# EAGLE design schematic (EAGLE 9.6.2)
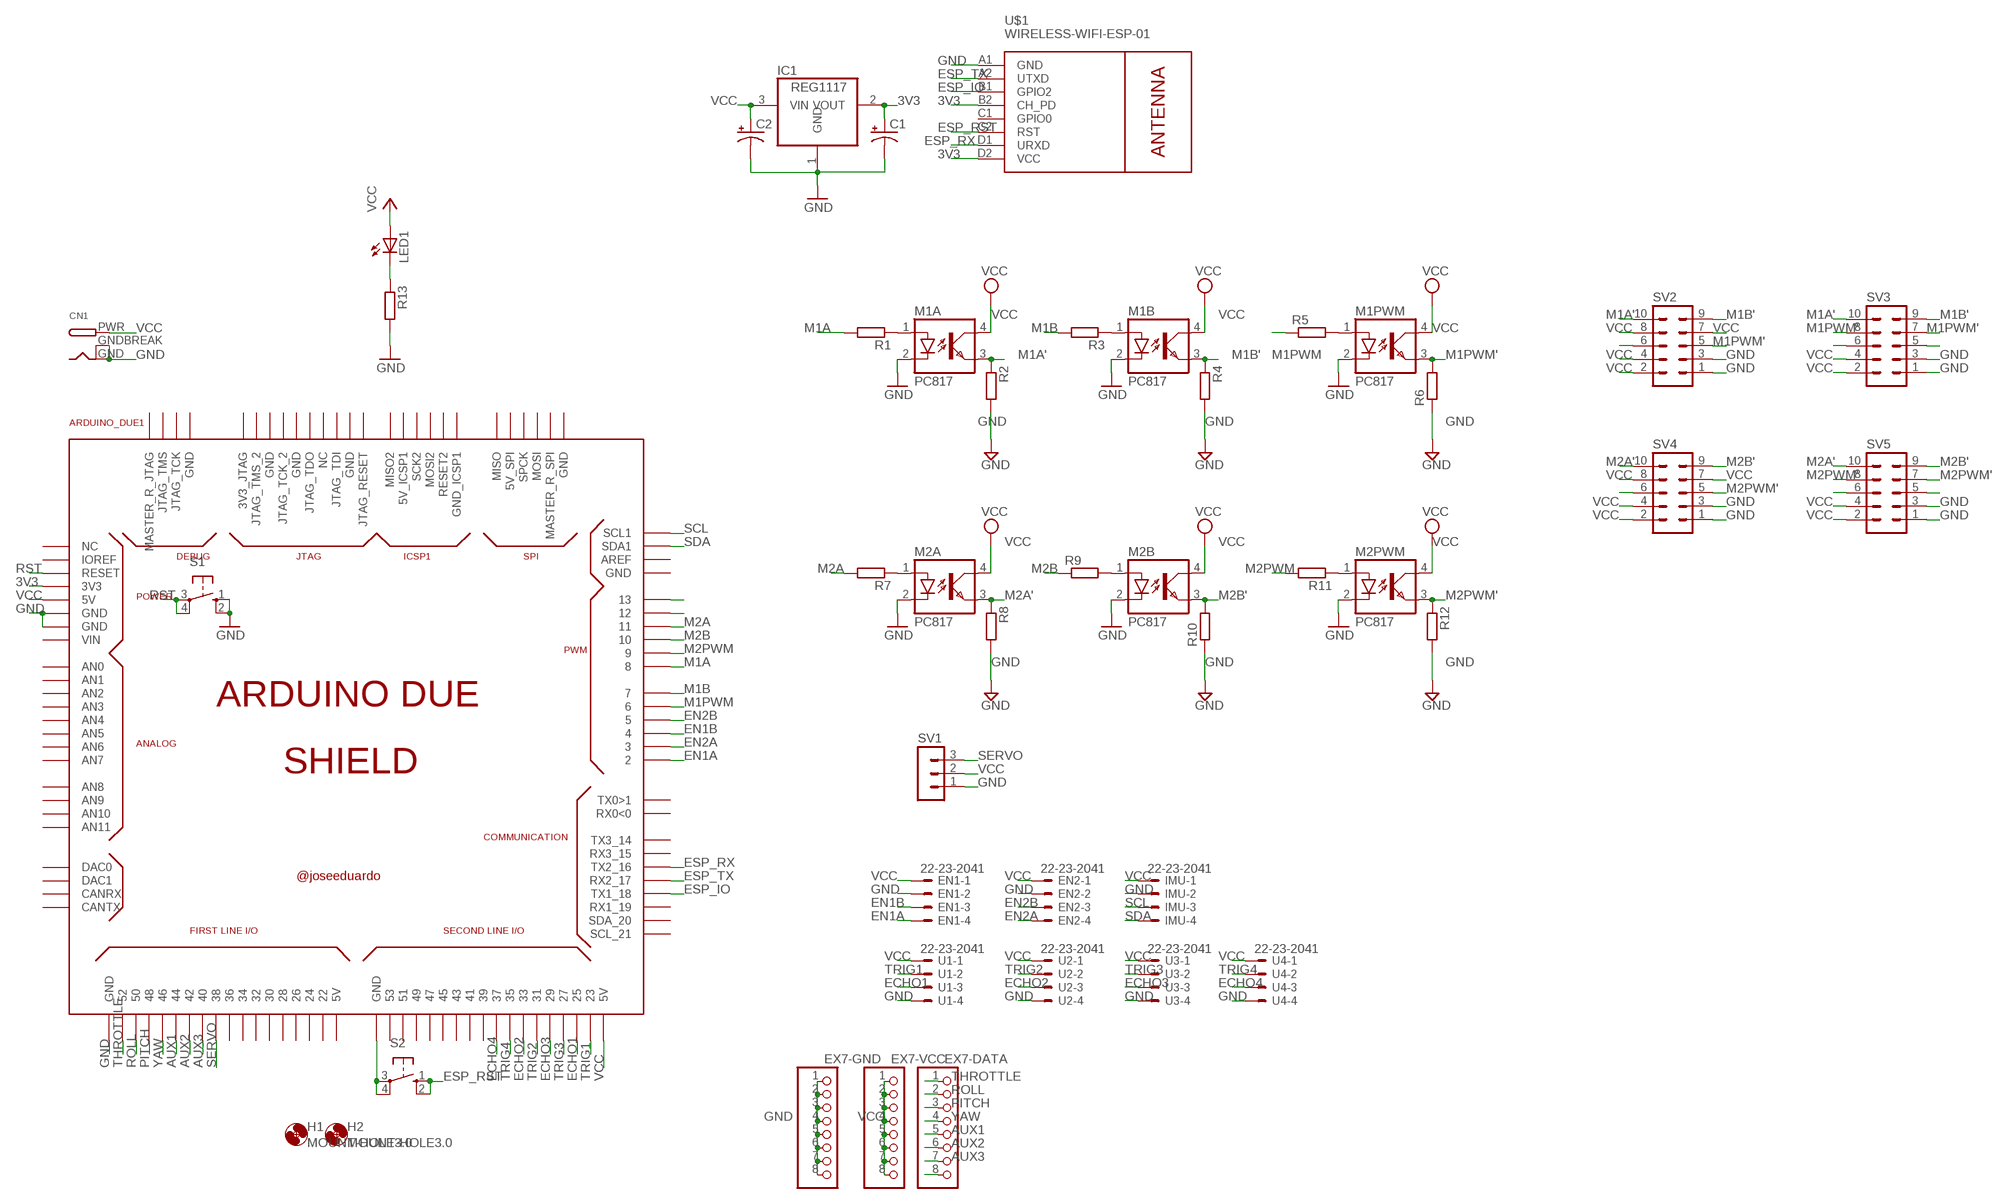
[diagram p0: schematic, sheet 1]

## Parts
ARDUINO_DUE1  ARDUINO_DUE_SHIELD  [ARDUINO_DUE_SHIELD]
C1  CPOL-USTT2D4  [TT2D4]
C2  CPOL-USTT2D4  [TT2D4]
CN1  DCBARRELPTH  [DCJACK_2MM_PTH]
EN1  22-23-2041  [22-23-2041]
EN2  22-23-2041  [22-23-2041]
EX7-DATA  PINHD-1X8BIG  [1X08-BIG]
EX7-GND  PINHD-1X8BIG  [1X08-BIG]
EX7-VCC  PINHD-1X8BIG  [1X08-BIG]
H1  MOUNT-HOLE3.0  [3,0]
H2  MOUNT-HOLE3.0  [3,0]
IC1  REG1117  [SOT223]
IMU  22-23-2041  [22-23-2041]
LED1  LED5MM  [LED5MM]
M1A  PC817  [DIL04]
M1B  PC817  [DIL04]
M1PWM  PC817  [DIL04]
M2A  PC817  [DIL04]
M2B  PC817  [DIL04]
M2PWM  PC817  [DIL04]
R1  R-EU_M0805  [M0805]
R2  R-EU_M0805  [M0805]
R3  R-EU_M0805  [M0805]
R4  R-EU_M0805  [M0805]
R5  R-EU_M0805  [M0805]
R6  R-EU_M0805  [M0805]
R7  R-EU_M0805  [M0805]
R8  R-EU_M0805  [M0805]
R9  R-EU_M0805  [M0805]
R10  R-EU_M0805  [M0805]
R11  R-EU_M0805  [M0805]
R12  R-EU_M0805  [M0805]
R13  R-EU_M0805  [M0805]
S1  40-XX  [B3F-40XX]
S2  40-XX  [B3F-40XX]
SV1  MA03-1  [MA03-1]
SV2  ML10  [ML10]
SV3  ML10  [ML10]
SV4  ML10  [ML10]
SV5  ML10  [ML10]
U1  22-23-2041  [22-23-2041]
U2  22-23-2041  [22-23-2041]
U3  22-23-2041  [22-23-2041]
U4  22-23-2041  [22-23-2041]
U$1  WIRELESS-WIFI-ESP-01  [WIRELESS-WIFI-ESP-01]

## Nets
3V3: ARDUINO_DUE1.3V3 C1.+ IC1.2(VOUT) U$1.B2(CH_PD) U$1.D2(VCC)
AUX1: ARDUINO_DUE1.44 EX7-DATA.5
AUX2: ARDUINO_DUE1.42 EX7-DATA.6
AUX3: ARDUINO_DUE1.40 EX7-DATA.7
ECHO1: ARDUINO_DUE1.25 U1.3
ECHO2: ARDUINO_DUE1.33 U2.3
ECHO3: ARDUINO_DUE1.29 U3.3
ECHO4: ARDUINO_DUE1.37 U4.3
EN1A: ARDUINO_DUE1.2 EN1.4
EN1B: ARDUINO_DUE1.4 EN1.3
EN2A: ARDUINO_DUE1.3 EN2.4
EN2B: ARDUINO_DUE1.5 EN2.3
ESP_IO: ARDUINO_DUE1.18(TX1_18) U$1.B1(GPIO2)
ESP_RST: S2.1(S) S2.2(S1) U$1.C2(RST)
ESP_RX: ARDUINO_DUE1.16(TX2_16) U$1.D1(URXD)
ESP_TX: ARDUINO_DUE1.17(RX2_17) U$1.A2(UTXD)
GND: ARDUINO_DUE1.GND ARDUINO_DUE1.GND_1(GND) ARDUINO_DUE1.GND_2(GND) C1.- C2.- CN1.GND CN1.GNDBREAK EN1.2 EN2.2 EX7-GND.1 EX7-GND.2 EX7-GND.3 EX7-GND.4 EX7-GND.5 EX7-GND.6 EX7-GND.7 EX7-GND.8 IC1.1(GND) IMU.2 M1A.2(C) M1B.2(C) M1PWM.2(C) M2A.2(C) M2B.2(C) M2PWM.2(C) R2.2 R4.2 R6.1 R8.2 R10.1 R12.2 R13.2 S1.1(S) S1.2(S1) SV1.1 SV2.1 SV2.3 SV3.1 SV3.3 SV4.1 SV4.3 SV5.1 SV5.3 U1.4 U2.4 U3.4 U4.4 U$1.A1(GND)
M1A: ARDUINO_DUE1.8 R1.2
M1A': M1A.3(EMIT) R2.1 SV2.10 SV3.10
M1B: ARDUINO_DUE1.7 R3.2
M1B': M1B.3(EMIT) R4.1 SV2.9 SV3.9
M1PWM: ARDUINO_DUE1.6 R5.1
M1PWM': M1PWM.3(EMIT) R6.2 SV2.5 SV3.7 SV3.8
M2A: ARDUINO_DUE1.11 R7.2
M2A': M2A.3(EMIT) R8.1 SV4.10 SV5.10
M2B: ARDUINO_DUE1.10 R9.1
M2B': M2B.3(EMIT) R10.2 SV4.9 SV5.9
M2PWM: ARDUINO_DUE1.9 R11.2
M2PWM': M2PWM.3(EMIT) R12.1 SV4.5 SV5.7 SV5.8
N$1: M1B.1(A) R3.1
N$2: M1A.1(A) R1.1
N$5: M1PWM.1(A) R5.2
N$6: SV2.6
N$7: M2A.1(A) R7.1
N$8: ARDUINO_DUE1.GND_3(GND) S2.3(P) S2.4(P1)
N$9: M2B.1(A) R9.2
N$10: EX7-DATA.8
N$11: M2PWM.1(A) R11.1
N$13: LED1.K(C) R13.1
N$16: ARDUINO_DUE1.12
N$21: ARDUINO_DUE1.13
N$23: SV3.6
N$28: SV3.5
N$33: SV4.6
N$42: SV5.6
N$48: SV5.5
PITCH: ARDUINO_DUE1.48 EX7-DATA.3
ROLL: ARDUINO_DUE1.50 EX7-DATA.2
RST: ARDUINO_DUE1.RESET S1.3(P) S1.4(P1)
SCL: ARDUINO_DUE1.SCL1 IMU.3
SDA: ARDUINO_DUE1.SDA1 IMU.4
SERVO: ARDUINO_DUE1.38 SV1.3
THROTTLE: ARDUINO_DUE1.52 EX7-DATA.1
TRIG1: ARDUINO_DUE1.23 U1.2
TRIG2: ARDUINO_DUE1.31 U2.2
TRIG3: ARDUINO_DUE1.27 U3.2
TRIG4: ARDUINO_DUE1.35 U4.2
VCC: ARDUINO_DUE1.5V0(5V) ARDUINO_DUE1.5V0_2(5V) C2.+ CN1.PWR EN1.1 EN2.1 EX7-VCC.1 EX7-VCC.2 EX7-VCC.3 EX7-VCC.4 EX7-VCC.5 EX7-VCC.6 EX7-VCC.7 EX7-VCC.8 IC1.3(VIN) IMU.1 LED1.A M1A.4(COL) M1B.4(COL) M1PWM.4(COL) M2A.4(COL) M2B.4(COL) M2PWM.4(COL) SV1.2 SV2.2 SV2.4 SV2.7 SV2.8 SV3.2 SV3.4 SV4.2 SV4.4 SV4.7 SV4.8 SV5.2 SV5.4 U1.1 U2.1 U3.1 U4.1
YAW: ARDUINO_DUE1.46 EX7-DATA.4
Unconnected: ARDUINO_DUE1.0(RX0<0) ARDUINO_DUE1.1(TX0>1) ARDUINO_DUE1.3V3_JTAG ARDUINO_DUE1.5V0_1(5V) ARDUINO_DUE1.5V_2(5V_SPI) ARDUINO_DUE1.5V_ICSP1 ARDUINO_DUE1.14(TX3_14) ARDUINO_DUE1.15(RX3_15) ARDUINO_DUE1.19(RX1_19) ARDUINO_DUE1.20(SDA_20) ARDUINO_DUE1.21(SCL_21) ARDUINO_DUE1.22 ARDUINO_DUE1.24 ARDUINO_DUE1.26 ARDUINO_DUE1.28 ARDUINO_DUE1.30 ARDUINO_DUE1.32 ARDUINO_DUE1.34 ARDUINO_DUE1.36 ARDUINO_DUE1.39 ARDUINO_DUE1.41 ARDUINO_DUE1.43 ARDUINO_DUE1.45 ARDUINO_DUE1.47 ARDUINO_DUE1.49 ARDUINO_DUE1.51 ARDUINO_DUE1.53 ARDUINO_DUE1.A0(AN0) ARDUINO_DUE1.A1(AN1) ARDUINO_DUE1.A2(AN2) ARDUINO_DUE1.A3(AN3) ARDUINO_DUE1.A4(AN4) ARDUINO_DUE1.A5(AN5) ARDUINO_DUE1.A6(AN6) ARDUINO_DUE1.A7(AN7) ARDUINO_DUE1.A8(AN8) ARDUINO_DUE1.A9(AN9) ARDUINO_DUE1.A10(AN10) ARDUINO_DUE1.A11(AN11) ARDUINO_DUE1.AREF ARDUINO_DUE1.CANRX ARDUINO_DUE1.CANTX ARDUINO_DUE1.DAC0 ARDUINO_DUE1.DAC1 ARDUINO_DUE1.GND_4(GND) ARDUINO_DUE1.GND_5(GND) ARDUINO_DUE1.GND_7(GND) ARDUINO_DUE1.GND_8(GND) ARDUINO_DUE1.GND_9(GND) ARDUINO_DUE1.GND_10(GND) ARDUINO_DUE1.GND_ICSP1 ARDUINO_DUE1.IOREF ARDUINO_DUE1.JTAG_RESET ARDUINO_DUE1.JTAG_TCK ARDUINO_DUE1.JTAG_TCK_2 ARDUINO_DUE1.JTAG_TDI ARDUINO_DUE1.JTAG_TDO ARDUINO_DUE1.JTAG_TMS ARDUINO_DUE1.JTAG_TMS_2 ARDUINO_DUE1.MASTER_RESET_JTAG(MASTER_R_JTAG) ARDUINO_DUE1.MASTER_RESET_SPI(MASTER_R_SPI) ARDUINO_DUE1.MISO ARDUINO_DUE1.MISO2 ARDUINO_DUE1.MOSI ARDUINO_DUE1.MOSI2 ARDUINO_DUE1.NC_2(NC) ARDUINO_DUE1.NC_5(NC) ARDUINO_DUE1.RESET2 ARDUINO_DUE1.SCK2 ARDUINO_DUE1.SPCK ARDUINO_DUE1.VIN U$1.C1(GPIO0)

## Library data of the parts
ARDUINO_DUE1 = arduino_due_shield:ARDUINO_DUE_SHIELD
C1 C2 = adafruit:CPOL-US: POLARIZED CAPACITOR, American symbol
CN1 = adafruit:DCBARREL: 2.0mm DC Barrel Jack DCJACK_2MM_PTH - Through Hole Jack (4UConnector: 05537)
EN1 EN2 IMU U1-U4 = con-molex:22-23-2041: .100" (2.54mm) Center Header - 4 Pin; MF: MOLEX; MPN: 22-23-2041; OC_FARNELL: 1462920; OC_NEWARK: 38C0355
EX7-DATA EX7-GND EX7-VCC = adafruit:PINHD-1X8: PIN HEADER
H1 H2 = holes:MOUNT-HOLE: MOUNTING HOLE with drill center marker
IC1 = burr-brown:REG1117: 800mA and 1A Low Dropout (LDO) Positive Regulator 1.8V, 2.5V, 2.85V, 3.3V, 5V, and Adj; MPN: REG1117; OC_FARNELL: 1097566; OC_NEWARK: 14P6981
LED1 = adafruit:LED: LED
M1A M1B M1PWM M2A M2B M2PWM = optocoupler:PC817: SHARP OPTO COUPLER; MPN: PC817X4J000F; OC_FARNELL: 9707727; OC_NEWARK: 97K7059
R1-R13 = rcl:R-EU_: RESISTOR, European symbol; SPICEPREFIX: R
S1 S2 = adafruit:40-XX: OMRON SWITCH; MF: OMRON COMPONENTS USA; MPN: B3F-4000; OC_FARNELL: 176434; OC_NEWARK: 36K3105
SV1 = con-lstb:MA03-1: PIN HEADER; OC_FARNELL: unknown; OC_NEWARK: unknown
SV2-SV5 = con-ml:ML10: HARTING; OC_FARNELL: unknown; OC_NEWARK: unknown
U$1 = ESP-01:WIRELESS-WIFI-ESP-01: Wireless Wi-Fi ESP-01 Module based on ESP8266 chip Click here to find device on ebay.com

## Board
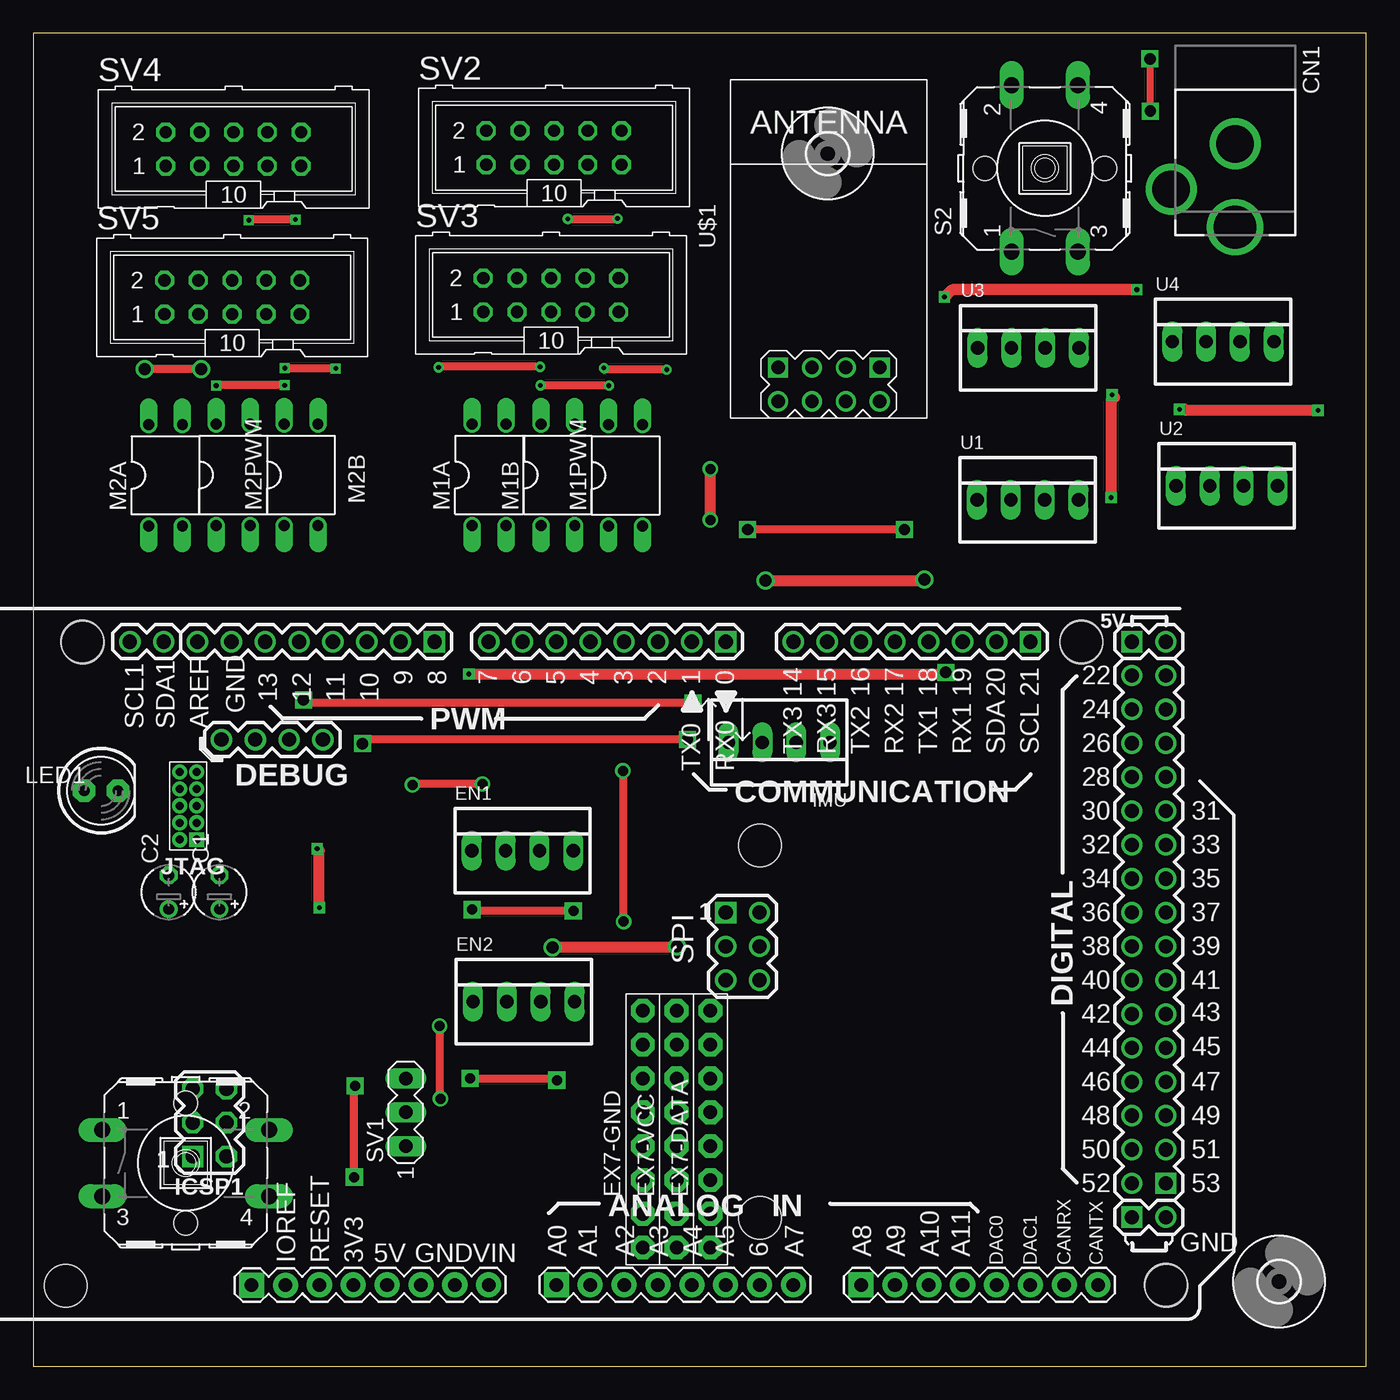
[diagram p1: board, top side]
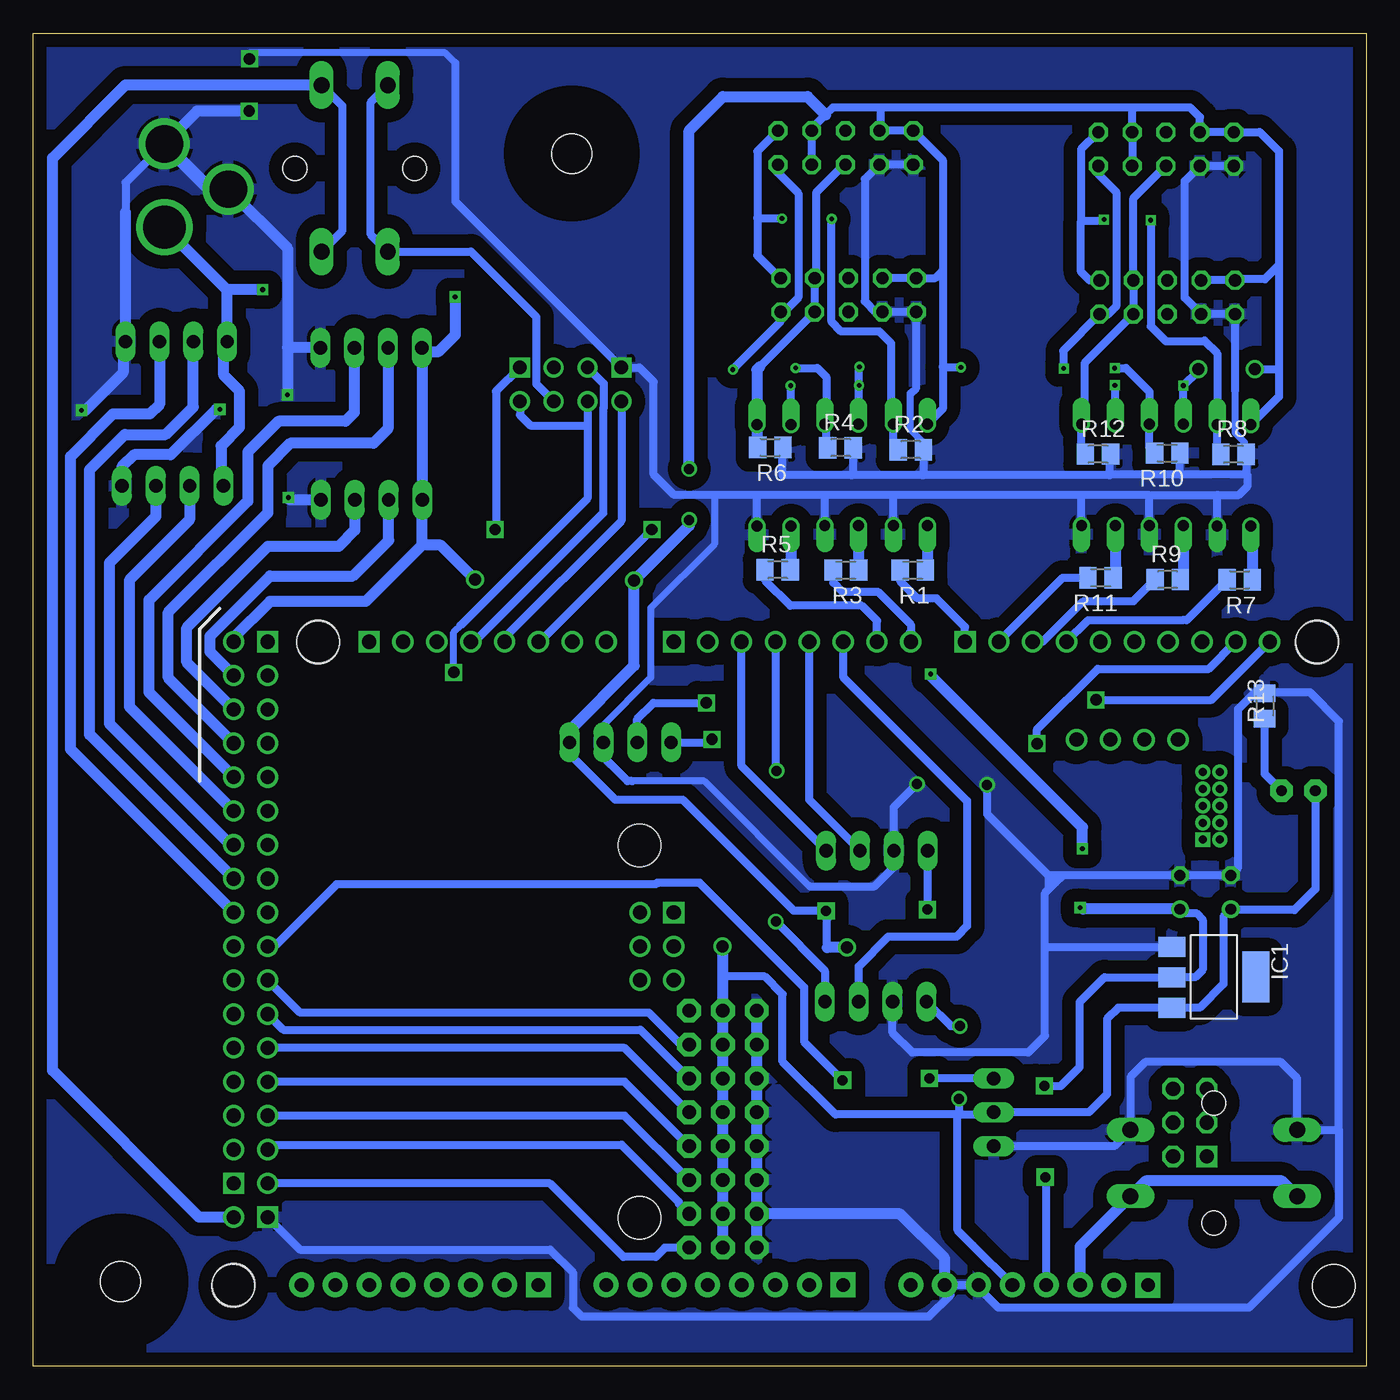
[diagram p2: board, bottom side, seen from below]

Size 100 x 100 mm. Coordinates in mm from the lower left corner, seen from the top.
Outline: 0,0 100,0 100,100 0,100 0,0
Copper layers (1*16): Top 0.035mm / dielectric 1.5mm / Bottom 0.035mm
Design rules "default": minimum track width 6mil, minimum drill 0.35mm, track to track 6mil, track to pad 6mil, pad to pad 6mil, via to via 6mil, smd to smd 6mil, copper to edge 40mil, drill to drill 6mil, minimum pad ring 10mil, minimum via ring 8mil, stop-mask expansion 4mil, vias tented up to drill 0mil, thermal gap 10mil

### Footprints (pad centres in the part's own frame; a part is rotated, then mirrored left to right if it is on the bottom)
ARDUINO_DUE_SHIELD = drill 1.067 square: 0 63.373,51.816; 5V0_1 93.853,51.816; 8 41.529,51.816; 21 86.233,51.816; 53 96.393,11.176; GND_2 93.853,8.636; MISO 63.373,31.496; MISO2 23.384,13.196 | drill 1.067: 1 60.833,51.816; 2 58.293,51.816; 3 55.753,51.816; 4 53.213,51.816; 5 50.673,51.816; 5V0_2 96.393,51.816; 5V_2 65.913,31.496; 6 48.133,51.816; 7 45.593,51.816; 9 38.989,51.816; 10 36.449,51.816; 11 33.909,51.816; 12 31.369,51.816; 13 28.829,51.816; 14 68.453,51.816; 15 70.993,51.816; 16 73.533,51.816; 17 76.073,51.816; 18 78.613,51.816; 19 81.153,51.816; 20 83.693,51.816; 22 93.853,49.276; 23 96.393,49.276; 24 93.853,46.736; 25 96.393,46.736; 26 93.853,44.196; 27 96.393,44.196; 28 93.853,41.656; 29 96.393,41.656; 30 93.853,39.116; 31 96.393,39.116; 32 93.853,36.576; 33 96.393,36.576; 34 93.853,34.036; 35 96.393,34.036; 36 93.853,31.496; 37 96.393,31.496; 38 93.853,28.956; 39 96.393,28.956; 40 93.853,26.416; 41 96.393,26.416; 42 93.853,23.876; 43 96.393,23.876; 44 93.853,21.336; 45 96.393,21.336; 46 93.853,18.796; 47 96.393,18.796; 48 93.853,16.256; 49 96.393,16.256; 50 93.853,13.716; 51 96.393,13.716; 52 93.853,11.176; AREF 23.749,51.816; GND_3 96.393,8.636; GND_4 26.289,51.816; GND_5 65.913,26.416; GND_7 33.161,44.473; JTAG_TCK 30.621,44.473; JTAG_TMS 28.081,44.473; MASTER_RESET_JTAG 25.541,44.473; MASTER_RESET_SPI 63.373,26.416; MOSI 65.913,28.956; SCL1 18.669,51.816; SDA1 21.209,51.816; SPCK 63.373,28.956 | drill 1.016 pad 1.88: 3V3 35.433,3.556; 5V0 37.973,3.556; A1 53.213,3.556; A2 55.753,3.556; A3 58.293,3.556; A4 60.833,3.556; A5 63.373,3.556; A6 65.913,3.556; A7 68.453,3.556; A9 76.073,3.556; A10 78.613,3.556; A11 81.153,3.556; CANRX 88.773,3.556; CANTX 91.313,3.556; DAC0 83.693,3.556; DAC1 86.233,3.556; GND 40.513,3.556; GND_1 43.053,3.556; IOREF 30.346,3.543; RESET 32.893,3.555; VIN 45.593,3.556 | drill 0.6 pad 1.016 square: 3V3_JTAG 23.689,36.964 | drill 1.067 octagon: 5V_ICSP1 25.924,13.196; GND_ICSP1 25.924,18.276; MOSI2 25.924,15.736; RESET2 23.384,18.276; SCK2 23.384,15.736 | drill 1.016 pad 1.88 square: A0 50.673,3.556; A8 73.533,3.556; NC_2 27.806,3.543 | drill 0.6 pad 1.143: GND_8 23.689,38.234; GND_9 23.689,40.774; GND_10 23.689,42.044; JTAG_RESET 22.419,42.044; JTAG_TCK_2 22.419,38.234; JTAG_TDI 22.419,40.774; JTAG_TDO 22.419,39.504; JTAG_TMS_2 22.419,36.964; NC_5 23.689,39.504 | hole 3.2: 15.113,51.816; 90.043,51.816; 96.393,3.556; 96.418,3.505; 15.138,51.765; 90.068,51.765; 13.868,3.505; 65.938,36.525; 65.938,8.585
TT2D4 = drill 0.813: + -1.27,0 | drill 0.813 octagon: - 1.27,0
DCJACK_2MM_PTH = drill 2.8: GND 0,7.35; GNDBREAK 4.8,10.75 | drill 3.2: PWR 0,13.6
22-23-2041 = drill 1 long: 1 -3.81,0; 2 -1.27,0; 3 1.27,0; 4 3.81,0
1X08-BIG = drill 1.016 pad 1.778 octagon: 1 -8.89,0; 2 -6.35,0; 3 -3.81,0; 4 -1.27,0; 5 1.27,0; 6 3.81,0; 7 6.35,0; 8 8.89,0
3,0 = hole 3: 0,0
SOT223 = smd 1.499 x 2.007: 1 -2.261,-3.15; 2 0.025,-3.15; 3 2.311,-3.15 | smd 3.81 x 2.007: 4 0,3.15
LED5MM = drill 0.813 pad 1.676 octagon: A -1.27,0; K 1.27,0
DIL04 = drill 0.813 offset: 1 -1.27,-3.81; 2 1.27,-3.81; 3 1.27,3.81; 4 -1.27,3.81
M0805 = smd 1.3 x 1.6: 1 -0.95,0; 2 0.95,0
B3F-40XX = drill 1.194 long: 1 -6.248,2.489; 2 6.248,2.489; 3 -6.248,-2.489; 4 6.248,-2.489 | hole 1.803: 0,-4.496; 0,4.496
MA03-1 = drill 1.016 long: 1 -2.54,0; 2 0,0; 3 2.54,0
ML10 = drill 0.914 octagon: 1 -5.08,-1.27; 2 -5.08,1.27; 3 -2.54,-1.27; 4 -2.54,1.27; 5 0,-1.27; 6 0,1.27; 7 2.54,-1.27; 8 2.54,1.27; 9 5.08,-1.27; 10 5.08,1.27
WIRELESS-WIFI-ESP-01 = drill 1 square: A1 -8.89,3.81; D1 -8.89,-3.81 | drill 1: A2 -11.43,3.81; B1 -8.89,1.27; B2 -11.43,1.27; C1 -8.89,-1.27; C2 -11.43,-1.27; D2 -11.43,-3.81

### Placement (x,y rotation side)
ARDUINO_DUE1  -11.43,2.54 0 top
C1  13.97,35.56 90 top
C2  10.16,35.56 90 top
CN1  90.17,99.06 180 top
EN1  36.71,38.68 0 top
EN2  36.8,27.35 0 top
EX7-DATA  50.8,17.78 90 top
EX7-GND  45.72,17.78 90 top
EX7-VCC  48.26,17.78 90 top
H1  93.46,6.35 0 top
H2  59.61,90.97 0 top
IC1  11.43,29.21 270 bottom
IMU  55.96,46.8 180 top
LED1  5.08,43.18 0 top
M1A  34.19,66.87 0 top
M1B  39.35,66.87 0 top
M1PWM  44.44,66.83 0 top
M2A  9.92,66.84 0 top
M2B  14.99,66.87 0 top
M2PWM  20.08,66.87 0 top
R1  34.02,59.73 180 bottom
R2  34.17,68.76 0 bottom
R3  39.04,59.73 180 bottom
R4  39.44,68.91 0 bottom
R5  44.15,59.75 0 bottom
R6  44.7,68.93 180 bottom
R7  9.5,58.99 180 bottom
R8  9.95,68.41 0 bottom
R9  14.9,59.02 0 bottom
R10  14.94,68.51 180 bottom
R11  19.93,59.16 180 bottom
R12  20.12,68.43 0 bottom
R13  7.62,49.53 90 bottom
S1  11.43,15.24 0 top
S2  75.89,89.87 90 top
SV1  27.94,19.05 90 top
SV2  39.06,91.42 0 top
SV3  38.84,80.37 0 top
SV4  15.02,91.32 0 top
SV5  14.92,80.19 0 top
U1  74.61,64.99 0 top
U2  89.54,66.04 0 top
U3  74.65,76.41 0 top
U4  89.27,76.87 0 top
U$1  59.69,83.82 90 top

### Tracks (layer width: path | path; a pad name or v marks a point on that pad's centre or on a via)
3V3  (via drill 0.35 pad 0.85, 0.75 pad 1.3, 0.85 pad 0.85)
  Top 0.61: v24.08,14.18 24.08,20.72 23.96,20.84 v24.14,21.02
  Top 0.813: v21.45,34.39 21.45,38.66 v21.29,38.82 | v21.29,38.82 | v32.68,51.93 68.56,51.93 68.57,51.95 v68.45,52.06
  Bottom 0.508: v68.45,52.06 68.45,55.08 67.96,55.57
  Bottom 0.61: C1.+ 13.67,33.99 12.76,33.99 12.26,33.49 12.26,29.75 12.82,29.18 IC1.2 19.63,29.18 21.5,27.32 21.5,22.44 22.91,21.02 v24.14,21.02 | U$1.D2 63.5,71.36 62.71,70.57 58.57,70.57 58.42,70.72 | ARDUINO_DUE1.3V3 24,14.1 v24.08,14.18 | 58.42,70.72 58.42,65.11 67.96,55.57 | U$1.B2 58.42,70.72
  Bottom 0.813: C1.+ 21.24,34.29 21.4,34.44 v21.45,34.39 | v21.29,38.82 21.29,40.44 32.68,51.83 v32.68,51.93
AUX1
  Bottom 0.61: EX7-DATA.5 55.63,23.88 ARDUINO_DUE1.44
AUX2
  Bottom 0.61: EX7-DATA.6 54.45,25.24 81.25,25.24 ARDUINO_DUE1.42
AUX3
  Bottom 0.61: EX7-DATA.7 51.44,24.13 53.82,26.51 79.98,26.51 ARDUINO_DUE1.40
ECHO1
  Bottom 0.813: ARDUINO_DUE1.25 88.49,52.81 88.49,55.42 82.4,61.51 77.09,61.51 75.88,62.72 U1.3
ECHO2
  Bottom 0.813: U2.3 90.81,63.76 94.3,60.27 94.3,48.22 85.2,39.12 ARDUINO_DUE1.33
ECHO3
  Bottom 0.813: ARDUINO_DUE1.29 91.31,50.54 91.31,57.49 83.92,64.89 83.92,68.58 81.61,70.89 76.58,70.89 75.92,71.55 U3.3
ECHO4
  Bottom 0.813: ARDUINO_DUE1.37 97.2,46.28 97.2,68.26 94.03,71.43 91.25,71.43 90.54,72.15 U4.3
EN1A
  Bottom 0.61: EN1.4 46.86,45.03 ARDUINO_DUE1.2
EN1B
  Bottom 0.61: EN1.3 41.78,42.49 ARDUINO_DUE1.4
EN2A  (via drill 0.75)
  Top 0.61: v44.23,44.66 44.23,33.42 v44.29,33.36
  Bottom 0.61: ARDUINO_DUE1.3 44.32,44.75 v44.23,44.66 | v44.29,33.36 40.61,29.67 EN2.4
EN2B
  Bottom 0.61: ARDUINO_DUE1.5 39.24,51.72 29.94,42.42 29.94,33.01 30.72,32.23 35.85,32.23 38.07,30.01 EN2.3
ESP_IO
  Bottom 0.61: U$1.B1 57.21,73.72 57.21,71.89 57.24,71.86 57.24,64 66.89,54.36 ARDUINO_DUE1.18
ESP_RST
  Bottom 0.61: U$1.C2 62.27,73.7 62.27,78.74 67.16,83.62 S2.1 74.69,84.91 74.69,94.83 S2.2
ESP_RX  (via drill 0.85 pad 0.85)
  Top 0.61: v65.35,62.77 54.02,62.77 53.96,62.83 53.65,62.83 v53.59,62.77
  Bottom 0.61: U$1.D1 65.29,73.14 65.29,62.83 v65.35,62.77 | v53.59,62.77 62,54.36 ARDUINO_DUE1.16
ESP_TX
  Bottom 0.61: U$1.A2 55.88,63.42 64.64,54.65 ARDUINO_DUE1.17
GND  (via drill 0.35 pad 0.85, 0.75, 0.85 pad 0.85)
  Top 0.508: v83.78,98.08 83.78,94.33 83.87,94.24 v83.81,94.17
  Top 0.61: v33.7,43.68 28.52,43.68 v28.45,43.61
  Top 0.813: v96.4,71.71 86.48,71.71 86.42,71.77 86.01,71.77 v85.99,71.78 | v80.88,65.17 80.88,72.45 81.12,72.69 | 81.12,72.69 | 81.12,72.69 v80.94,72.88
  Bottom 0.152: 36.39,79.1 SV3.3
  Bottom 0.508: 48.91,65.36 48.91,61.65 53.67,56.88 53.67,51.66 57.23,48.1 IMU.2 | 41.75,36.01 49.65,43.9 55.07,43.9 | 68.34,97.79 69.09,98.53 83.78,98.53 v83.78,98.08 | R2.2 33.22,69.3 34.2,70.27 34.2,72.96 34.18,72.98 | 9.84,73.2 9.84,70.03 9.13,69.32 9.13,68.54 R8.2
  Bottom 0.61: 7.99,50.48 8.44,50.48 9.6,49.32 9.6,37.39 C2.- C1.- 22.77,36.83 | 7.99,50.48 R13.2 | SV1.1 18.9,16.51 S1.2 17.68,21.7 16.57,22.81 6.41,22.81 5.18,21.59 S1.1 2.04,17.73 | ARDUINO_DUE1.GND_1 31.19,6.1 | 31.19,6.1 ARDUINO_DUE1.GND 29.08,5.89 27.61,4.42 8.78,4.42 2.03,11.16 2.03,17.72 2.04,17.73 | 2.04,17.73 2.04,48.39 4.2,50.55 7.92,50.55 7.99,50.48 | IC1.1 24.06,31.47 24.1,31.51 | ARDUINO_DUE1.GND_2 80,8.75 61.21,8.75 59.51,7.04 59.51,4.38 58.87,3.73 32.79,3.73 31.19,5.33 31.19,6.1 | 24.1,31.51 24.1,24.8 25.36,23.54 34.06,23.54 35.53,25.01 EN2.2 | 24.1,31.51 24.1,35.5 23.85,35.75 | 23.85,35.75 23.31,36.29 | 23.31,36.29 22.77,36.83 | M2A.2 11.19,65.34 11.16,65.36 | 16.36,65.36 11.16,65.36 | 16.36,65.36 21.42,65.36 | 21.42,65.36 35.33,65.36 | 35.33,65.36 40.65,65.36 | 40.65,65.36 45.71,65.36 | M1PWM.2 45.71,65.36 | M2B.2 16.26,65.26 16.36,65.36 | M2PWM.2 21.35,65.3 21.42,65.36 | M1A.2 35.46,65.23 35.33,65.36 | M1B.2 40.62,65.34 40.65,65.36 | 45.71,65.36 48.91,65.36 51.93,65.36 53.47,66.9 53.47,73.87 54.53,74.93 U$1.A1 68.34,87.39 68.34,97.79 | CN1.GND 90.41,91.47 93.08,88.8 93.08,86.55 | 55.07,43.9 55.43,43.9 57.23,45.71 IMU.2 | R8.2 9,66.96 | 9,66.96 9.09,66.88 13.87,66.88 | R10.1 13.99,67 13.87,66.88 | 13.87,66.88 19.18,66.88 19.24,66.82 19.24,66.85 | 19.24,66.85 19.24,68.35 R12.2 | 19.24,66.85 33.27,66.85 | 33.27,66.85 33.25,66.82 33.22,66.85 R2.2 | 33.27,66.85 38.61,66.85 | 38.61,66.85 43.73,66.85 43.78,66.8 43.78,68.9 R6.1 | R4.2 38.49,66.96 38.61,66.85 | SV3.3 SV3.1 33.76,73.4 34.18,72.98 | SV2.1 SV2.3 37.61,89.07 37.61,79.9 36.8,79.1 36.39,79.1 | SV4.1 SV4.3 13.61,88.91 13.61,80.16 SV5.3 SV5.1 9.84,73.2
  Bottom 0.61: 11.16,65.36 9.57,65.36 8.89,66.04 8.89,66.85 9,66.96 | 41.75,36.01 36.88,36.01 35.44,37.44 EN1.2 35.44,41.95 v33.7,43.68 | v28.45,43.61 28.45,41.43 23.85,36.83 | 23.85,36.83 23.31,36.29 | 22.77,36.83 23.85,36.83 | 23.85,36.83 23.85,35.75
  Bottom 0.813: U2.4 93.35,67.48 92.45,68.39 89.7,68.39 86.3,71.78 v85.99,71.78 | v96.4,71.71 96.09,71.71 93.26,74.53 93.26,76.69 U4.4 93.08,86.55 | U1.4 80.76,64.99 80.88,65.11 v80.88,65.17 | CN1.GNDBREAK 80.94,83.88 80.94,76.46 | 80.94,76.46 v80.94,72.88 | U3.4 80.89,76.41 80.94,76.46 | v83.81,94.17 87.71,94.17 90.41,91.47 | EX7-GND.1 EX7-GND.2 | EX7-GND.2 EX7-GND.3 EX7-GND.4 EX7-GND.5 EX7-GND.6 EX7-GND.7 EX7-GND.8 | ARDUINO_DUE1.GND_1 31.62,8.09 34.97,11.43 EX7-GND.2
  Bottom 1.016: CN1.GND 86.77,88.31 CN1.GNDBREAK
  pour Bottom (isolate 1.016): 0,99.06 0,0 100.33,0 100.33,100.33 0,100.33
M1A
  Bottom 0.61: R1.2 34.97,58.92 33.65,57.6 32.23,57.6 30.1,55.47 ARDUINO_DUE1.8
M1A'  (via drill 0.35)
  Top 0.61: v40.1,86.07 43.78,86.07 43.81,86.1 v43.84,86.1
  Bottom 0.152: SV2.10 44.33,92.5
  Bottom 0.61: 45.68,86.16 45.68,91.16 44.33,92.5 | 45.68,86.16 45.68,83.33 43.99,81.64 SV3.10 | v43.84,86.1 45.62,86.1 45.68,86.16 | v40.1,86.07 40.12,86.06 40.12,78.36 39.39,77.63 36.52,77.63 35.63,76.73 35.63,70.85 M1A.3 35.46,69.09 R2.1
M1B
  Bottom 0.61: R3.2 39.99,58.78 39.32,58.11 36.64,58.11 34.16,55.63 34.16,54.94
  Bottom 0.813: 34.16,54.94 ARDUINO_DUE1.7
M1B'  (via drill 0.35)
  Top 0.61: v47.52,74.77 42.85,74.77 42.77,74.85 v42.81,74.89
  Bottom 0.152: 43.53,79.24 43.67,79.1 SV3.9
  Bottom 0.61: 43.53,79.24 42.6,80.17 42.6,87.99 44.14,89.54 SV2.9 | SV3.9 43.92,78.42 47.52,74.82 v47.52,74.77 | v42.81,74.89 41.19,74.89 40.5,74.21 40.5,70.8 | 40.5,70.8 M1B.3 | R4.1 40.5,69.02 40.5,70.8
M1PWM
  Bottom 0.61: R5.1 45.1,58.96 43.21,57.06 37.84,57.06 36.7,55.93 ARDUINO_DUE1.6
M1PWM'
  Bottom 0.152: 41.41,81.66 SV3.8 41.38,81.94
  Bottom 0.61: SV3.8 SV3.7 45.48,74.99 | SV2.5 39.16,90.16 41.28,88.04 41.28,82.05 41.38,81.94
  Bottom 0.813: 45.48,74.99 45.71,74.77 45.71,71.14 | 45.71,71.14 M1PWM.3 | R6.2 45.65,71.08 45.71,71.14
M2A
  Bottom 0.61: ARDUINO_DUE1.11 20.86,55.98 13.78,55.98 13.46,55.98 R7.2
M2A'  (via drill 0.35)
  Top 0.61: v19.68,86.03 16.17,86.03 v16.17,85.99
  Bottom 0.152: 20.04,81.47 SV5.10
  Bottom 0.61: SV4.10 21.4,91.29 21.4,85.9 | 21.4,85.9 21.4,82.11 20.76,81.47 20.04,81.47 | 21.4,85.9 21.36,85.94 19.74,85.94 19.68,86.01 v19.68,86.03 | v16.17,85.99 16.17,78.03 15.03,76.89 12.2,76.89 12.13,76.95 11.19,76 M2A.3 11.19,68.69 R8.1
M2B
  Bottom 0.61: R9.1 17.46,57.4 21.21,57.4 24.26,54.36 ARDUINO_DUE1.10
M2B'  (via drill 0.35)
  Top 0.61: v22.69,74.85 18.9,74.85 v18.86,74.89
  Bottom 0.152: 18.94,79.33 18.88,79.39
  Bottom 0.61: 18.88,79.39 18.75,79.53 18.75,88.08 20.1,89.44 SV4.9 | 18.94,79.33 19.35,78.92 SV5.9 22.74,76.19 22.74,74.82 22.69,74.82 v22.69,74.85 | v18.86,74.89 18.03,74.89 16.26,73.11 M2B.3 16.26,68.88 R10.2
M2PWM
  Bottom 0.61: ARDUINO_DUE1.9 22.76,59.16 R11.2
M2PWM'
  Bottom 0.61: SV4.5 15.06,90.05 17.46,87.64 SV5.8 SV5.7 21.13,75.26 21.13,70.9 M2PWM.3 21.35,68.7 R12.1
N$1
  Bottom 0.813: M1B.1 38.08,60.03 38.09,60.02 R3.1
N$2
  Bottom 0.813: M1A.1 32.92,59.9 33.07,59.75 R1.1
N$5
  Bottom 0.813: M1PWM.1 43.17,60.49 R5.2
N$7
  Bottom 0.813: M2A.1 8.56,62.95 8.56,59 R7.1
N$8
  Bottom 0.61: S2.4 76.8,94.53 76.8,85.2 S2.3
  Bottom 0.813: 78.32,96.06 S2.4 93.09,96.12 98.56,90.65 98.56,22.18 87.56,11.18 ARDUINO_DUE1.GND_3
N$9
  Bottom 0.813: M2B.1 13.72,59.24 R9.2
N$11
  Bottom 0.813: M2PWM.1 18.81,59.32 R11.1
N$13
  Bottom 0.61: LED1.K 7.62,44.45 R13.1
PITCH
  Bottom 0.61: EX7-DATA.3 55.63,18.8 ARDUINO_DUE1.48
ROLL
  Bottom 0.61: EX7-DATA.2 51.59,12.22 51.59,12.34 55.86,16.61 82.07,16.61 ARDUINO_DUE1.50
RST
  Bottom 0.813: S1.3 6.33,13.89 16.54,13.89 S1.4 21.46,8.97 ARDUINO_DUE1.RESET
SCL  (via drill 0.85 pad 0.85)
  Top 0.61: v49.5,49.77 20.4,49.77 20.23,49.95 v20.27,49.99
  Bottom 0.61: IMU.3 54.69,48.55 53.47,49.77 v49.5,49.77 | v20.27,49.99 11.6,49.99 ARDUINO_DUE1.SCL1
SDA  (via drill 0.85 pad 0.85)
  Top 0.61: v49.08,47.03 24.8,47.03 24.59,46.81 v24.7,46.71
  Bottom 0.61: IMU.4 48.88,46.8 48.86,46.81 v49.08,47.03 | v24.7,46.71 24.7,47.78 20.15,52.33 11.81,52.33 ARDUINO_DUE1.SDA1
SERVO  (via drill 0.75 pad 1.3)
  Top 0.61: v32.77,21.6 38.96,21.6 39.05,21.68 v39.28,21.45
  Bottom 0.61: SV1.3 v32.77,21.59 v32.77,21.6 | v39.28,21.45 42.17,24.34 42.17,28.43 50.01,36.27 53.17,36.27 53.3,36.14 77.25,36.14 81.89,31.5 ARDUINO_DUE1.38
THROTTLE
  Bottom 0.61: EX7-DATA.1 52.61,8.89 53.3,8.2 55.72,8.2 61.23,13.72 ARDUINO_DUE1.52
TRIG1
  Bottom 0.813: U1.2 73.34,61.96 76.02,59.28 82.23,59.28 86.74,54.78 86.74,53.59 ARDUINO_DUE1.23
TRIG2
  Bottom 0.813: ARDUINO_DUE1.31 92.8,49.49 92.8,58.97 88.27,63.5 U2.2
TRIG3
  Bottom 0.813: ARDUINO_DUE1.27 89.86,51.64 89.86,56.56 82.42,64.01 82.42,67.54 80.71,69.24 74.47,69.24 73.38,70.33 U3.2
TRIG4
  Bottom 0.813: ARDUINO_DUE1.35 95.78,47.39 95.78,67.25 93.13,69.9 90.07,69.9 88,71.97 U4.2
VCC  (via drill 0.35, 0.35 pad 0.85, 0.75, 0.75 pad 1.3, 0.9)
  Top 0.61: v32.92,34.26 33.02,34.16 v40.52,34.16 | v43.18,73.56 38.1,73.56 38.06,73.61 v38.05,73.59 | v38.02,74.98 30.41,74.98 v30.41,74.94 | v18.86,73.59 13.87,73.59 13.81,73.66 v13.72,73.56 | v12.61,74.82 v8.36,74.82 | v30.48,25.52 30.48,20.12 v30.54,20.06
  Top 0.813: v82.8,80.77 | v82.8,80.77 68.9,80.77 v68.35,80.21 | v48.28,31.51 48.17,31.4 v38.96,31.4 | v54.92,58.94 66.78,58.94 v66.87,59.03 | v50.8,63.5 v50.8,67.31
  Bottom 0.152: SV4.2 9.57,92.58 | 31.77,82.24 31.77,82.2 31.83,82.13 | 32.33,81.64 34.11,81.64
  Bottom 0.61: LED1.A 3.81,35.79 5.39,34.21 10.08,34.21 C2.+ 10.71,33.74 10.71,28.68 12.49,26.9 IC1.3 18.6,26.9 19.45,26.05 19.45,20.39 20.8,19.05 SV1.2 28.11,18.88 30.65,18.88 | 40.45,31.4 40.45,33.53 40.52,33.59 v40.52,34.16 42.94,34.16 51.26,42.48 56.33,42.48 59.97,46.12 59.97,46.8 IMU.1 | EN1.1 32.92,38.66 v32.92,34.26 | ARDUINO_DUE1.5V0 29.5,9.05 30.65,10.2 30.65,18.88 | SV3.4 34.11,81.64 SV3.2 32.33,81.64 31.83,82.13 | SV2.7 SV2.8 41.68,92.77 40.55,93.89 40.02,94.43 36.39,94.43 | SV4.8 SV4.7 | SV5.4 SV5.2 9.76,81.55 7.6,81.55 6.55,82.6 | 17.65,92.67 SV4.8 | 6.55,82.6 6.55,91.16 7.98,92.58 SV4.2 SV4.4 12.48,93.71 13.2,94.43 17.4,94.43 | 6.55,82.6 6.55,74.82 | 6.55,74.82 6.55,72.74 M2A.4 | 31.77,74.98 31.77,82.24 31.77,90.48 SV2.2 SV2.4 36.39,92.83 36.39,94.43 | 31.77,74.98 31.77,71.83 M1A.4 | M1B.4 38.08,73.59 v38.05,73.59 38.05,74.83 38.06,74.85 38.06,74.94 v38.02,74.98 | M1PWM.4 43.17,73.52 43.15,73.54 v43.18,73.56 | v30.41,74.94 31.73,74.94 31.77,74.98 | 17.4,94.43 36.39,94.43 | SV4.8 17.56,94.27 17.4,94.43 | M2PWM.4 18.81,73.37 18.86,73.42 v18.86,73.59 | M2B.4 v13.72,73.56 12.61,74.67 v12.61,74.82 | v8.36,74.82 6.55,74.82 | EN2.1 31.17,25.52 v30.48,25.52 | v30.54,20.06 30.54,18.98 30.65,18.88 | 48.26,29.23 45.11,29.23 43.78,27.9 43.78,22.85 39.81,18.88 30.65,18.88
  Bottom 0.813: 70.84,65.03 U3.1 70.52,76.08 69.64,76.08 68.35,77.37 v68.35,80.21 | 70.84,65.03 U1.1 | U2.1 85.92,66.23 85.92,69.05 84.52,70.44 84.52,73.15 85.71,74.34 85.71,77.13 U4.1 85.46,80.75 85.48,80.77 | v82.8,80.77 85.48,80.77 | 85.48,80.77 CN1.PWR | ARDUINO_DUE1.5V0_2 84.96,54.65 82.24,57.38 75.06,57.38 70.84,61.59 | EX7-VCC.1 EX7-VCC.2 EX7-VCC.3 EX7-VCC.4 EX7-VCC.5 EX7-VCC.6 EX7-VCC.7 EX7-VCC.8 48.26,29.23 48.26,31.49 v48.28,31.51 | 40.45,31.4 | v38.96,31.4 40.45,31.4 | 70.84,61.59 70.84,65.03 | IMU.1 59.77,47.7 54.92,52.56 v54.92,58.94 50.8,63.06 v50.8,63.5 | v66.87,59.03 69.44,61.59 70.84,61.59 | v50.8,67.31 50.8,92.71 48.26,95.25 41.91,95.25 40.55,93.89
YAW
  Bottom 0.61: EX7-DATA.4 55.63,21.34 ARDUINO_DUE1.46

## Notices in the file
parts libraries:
ESP-01: Released under the Creative Commons Attribution 4.0 International License: http://creativecommons.org/licenses/by/4.0
